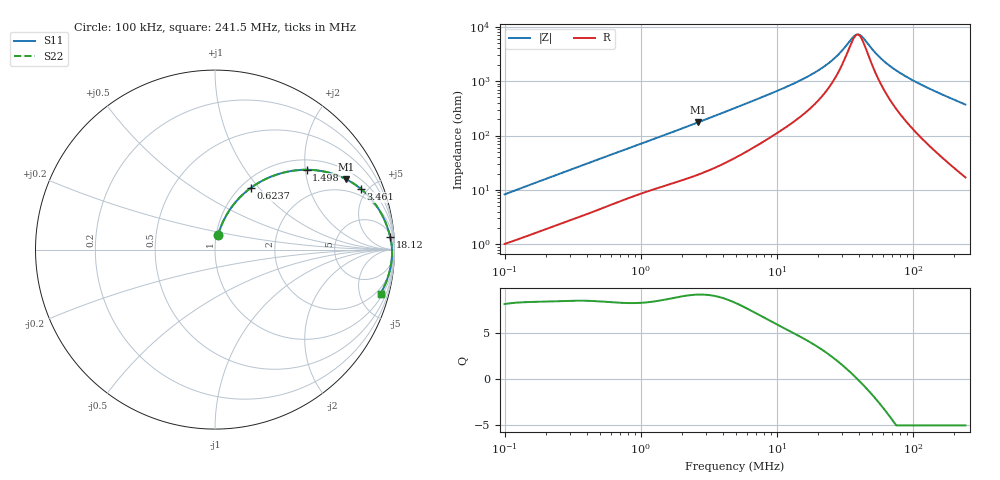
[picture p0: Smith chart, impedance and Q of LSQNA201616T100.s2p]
! LSQNA201616T100  S-PARAMETER MODEL  ( General Type )
! Model Generated by TAIYO YUDEN Corporation (http://www.ty-top.com)
! Version 2.0
! TAIYO YUDEN Control No. 100810NF25SB-FKC
! Copyright(c) 2007 TAIYO YUDEN CO.,LTD. All Rights Reserved.
! Product Description (link to TY-COMPAS)
! https://ds.yuden.co.jp/TYCOMPAS/or/detail?pn=LSQNA201616T100K&u=M
! Products Name : Inductors
! Characteristics :
!  Inductance : 10 uH , SRF(min) : 32 MHz , DC Resistance(max) : 0.65 Ohm
!  Rated Current : Saturation :250 mA , Temp Rise : 520 mA (40 degC)
!  Case Size : 2.0 x 1.6 / 0.079 x 0.063 [mm/inch] , Thickness : 1.6 / 0.063 [mm/inch]
!  (Conditions: Temperature = 25 degC , DC Bias Current/Voltage = 0A / 0V)
! External Node Assignments :
!  1  o---GGG---o  2
! GND o---------o GND
! Frequency Range : 0.1MHz  -  241.513628MHz  [ 402 STEP ]
# MHz S RI R 50
! Freq[MHz].  S11 Real  S11 Imag  S21 Real  S21 Imag  S12 Real  S12 Imag  S22 Real  S22 Imag
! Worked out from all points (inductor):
!   401 points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, 100 kHz to 241.5 MHz, reference 50 ohm
!   read as one part in series: L = 12.9 uH near 104 kHz
!   highest Q = 9.1 at 2.635 MHz (marker M1), where L = 10.5 uH
!   self-resonance near 38.94 MHz
!   S11 on the Smith chart (normalised r, x): 100 kHz: 1.02, +0.16; 623.7 kHz: 1.11, +0.91; 1.498 MHz: 1.24, +2.03; 3.461 MHz: 1.50, +4.52; 18.12 MHz: 8, +26; 241.5 MHz: 1.34, -7.42
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0.1  0.0166 0.08  0.9834 -0.08  0.9834 -0.08  0.0166 0.08
0.193888  0.0398 0.1446  0.9602 -0.1446  0.9602 -0.1446  0.0398 0.1446
0.368674  0.0978 0.2437  0.9022 -0.2437  0.9022 -0.2437  0.0978 0.2437
0.623722  0.2003 0.3443  0.7997 -0.3443  0.7997 -0.3443  0.2003 0.3443
0.902986  0.3129 0.4066  0.6871 -0.4066  0.6871 -0.4066  0.3129 0.4066
1.359207  0.4703 0.4434  0.5297 -0.4434  0.5297 -0.4434  0.4703 0.4434
1.498208  0.5107 0.4448  0.4893 -0.4448  0.4893 -0.4448  0.5107 0.4448
2.635333  0.7316 0.3916  0.2684 -0.3916  0.2684 -0.3916  0.7316 0.3916
3.461294  0.8127 0.3384  0.1873 -0.3384  0.1873 -0.3384  0.8127 0.3384
4.914404  0.8851 0.2638  0.1149 -0.2638  0.1149 -0.2638  0.8851 0.2638
10.7094  0.9585 0.1298  0.0415 -0.1298  0.0415 -0.1298  0.9585 0.1298
18.11814  0.9768 0.0688  0.0232 -0.0688  0.0232 -0.0688  0.9768 0.0688
25.72444  0.983 0.0358  0.017 -0.0358  0.017 -0.0358  0.983 0.0358
29.48135  0.9845 0.0238  0.0155 -0.0238  0.0155 -0.0238  0.9845 0.0238
35.81962  0.986 0.00713  0.014 -0.00713  0.014 -0.00713  0.986 0.00713
38.72134  0.9863 0.000475  0.0137 -0.000475  0.0137 -0.000475  0.9863 0.000475
41.85813  0.9865 -0.0062  0.0135 0.0062  0.0135 0.0062  0.9865 -0.0062
53.91696  0.9864 -0.0285  0.0136 0.0285  0.0136 0.0285  0.9864 -0.0285
66.79689  0.9851 -0.0488  0.0149 0.0488  0.0149 0.0488  0.9851 -0.0488
84.38097  0.9823 -0.0735  0.0177 0.0735  0.0177 0.0735  0.9823 -0.0735
110.8275  0.9762 -0.1069  0.0238 0.1069  0.0238 0.1069  0.9762 -0.1069
241.5136  0.9227 -0.2451  0.0773 0.2451  0.0773 0.2451  0.9227 -0.2451
